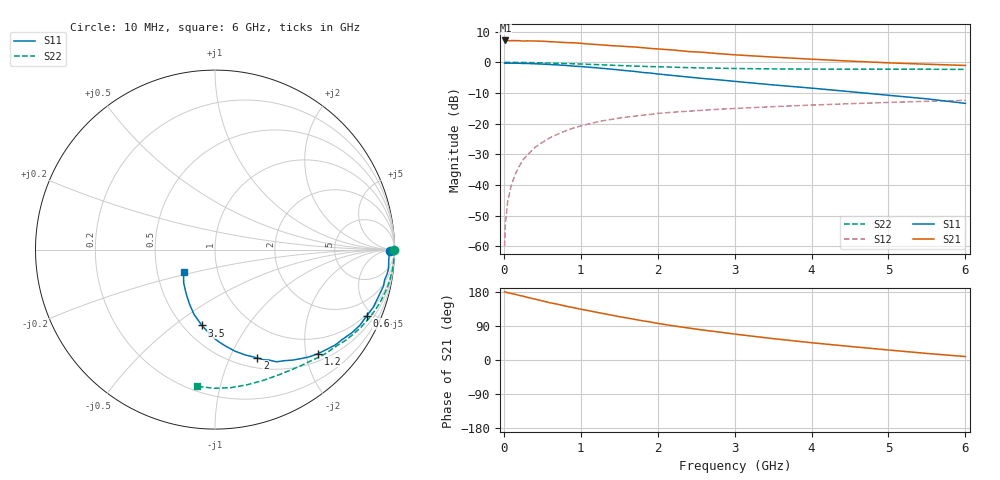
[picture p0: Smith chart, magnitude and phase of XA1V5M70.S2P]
! SIEMENS Discrete & RF Semiconductors
! BFY180
! Si NPN RF Bipolar Junction Transistor in MICRO-X
! VCE = 1.5 V  IC = 0.7 mA
! Common Emitter S-Parameters:  May  1997
# GHz  S  MA  R  50
!  f  S11  S21  S12  S22
! GHz  MAG  ANG  MAG  ANG  MAG  ANG  MAG  ANG
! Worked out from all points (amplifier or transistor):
!   36 points, 10 MHz to 6 GHz, reference 50 ohm
!   highest |S21| = 7.2 dB at 20 MHz (marker M1)
!   |S21| within 3 dB of that: start of sweep to 2.134 GHz
!   unconditionally stable (mu >= 1): 4.085 GHz to end of sweep
!   at 250 MHz: K = 0.05, MSG = 19.4 dB, |S12| = -31.8 dB
!   at 1.4 GHz: K = 0.47, MSG = 12.0 dB, |S12| = -18.6 dB
!   at 6 GHz: K = 1.07, MAG = 4.1 dB, |S12| = -12.4 dB
!   S11 on the Smith chart (normalised r, x): 10 MHz: 70, -13; 600 MHz: 0.93, -4.61; 1.2 GHz: 0.65, -2.25; 2 GHz: 0.61, -1.27; 3.5 GHz: 0.61, -0.64; 6 GHz: 0.68, -0.18
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0.01  0.9728 -0.3  2.249 179.8  0.001 82.7  0.9992 -0.2
0.02  0.967 -0.8  2.28 179.0  0.0023 97.4  0.9999 -0.5
0.05  0.9705 -2.0  2.264 177.7  0.0054 84.9  0.9988 -1.2
0.1  0.9702 -4.0  2.265 175.4  0.0102 87.1  0.9972 -2.6
0.2  0.969 -8.0  2.259 170.5  0.0201 84.5  0.9959 -5.1
0.25  0.9596 -10.2  2.227 168.4  0.0257 83.9  0.9963 -6.3
0.4  0.9484 -15.8  2.234 160.9  0.0405 78.6  0.9888 -10.0
0.6  0.9226 -23.6  2.178 151.0  0.0588 72.5  0.9749 -14.9
0.9  0.8704 -34.8  2.092 138.3  0.0844 64.1  0.9489 -21.8
1.1  0.8356 -41.6  1.995 130.2  0.0986 59.3  0.9293 -26.0
1.2  0.8164 -45.2  1.957 126.1  0.1057 56.9  0.9205 -28.2
1.5  0.7525 -54.9  1.848 114.4  0.1232 50.6  0.8906 -33.9
1.7  0.7127 -61.3  1.784 107.3  0.1324 47.0  0.8687 -37.4
2  0.6473 -68.7  1.658 96.6  0.1467 42.0  0.8488 -42.4
2.2  0.6106 -74.0  1.593 90.3  0.1539 38.8  0.8353 -45.6
2.6  0.5442 -83.2  1.458 78.7  0.166 33.9  0.811 -51.3
3  0.49 -91.2  1.33 68.4  0.1768 29.3  0.7953 -56.8
3.5  0.429 -99.8  1.22 56.4  0.1894 24.7  0.7828 -63.2
4  0.3799 -107.9  1.128 45.6  0.201 20.0  0.7767 -69.8
4.5  0.3329 -115.5  1.049 35.8  0.2117 15.8  0.774 -76.5
5.5  0.2541 -133.4  0.933 17.3  0.2317 7.4  0.7728 -90.4
6  0.2142 -144.8  0.891 9.1  0.2399 3.0  0.7683 -97.4
